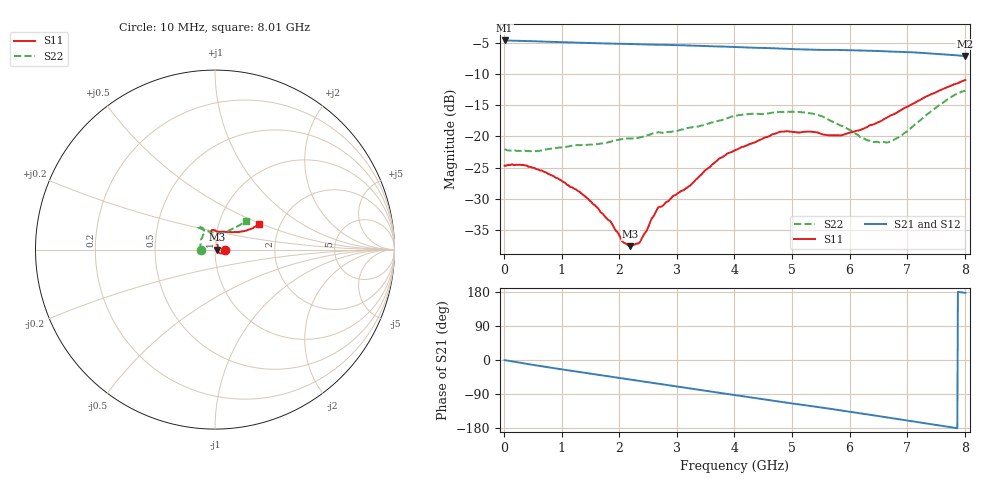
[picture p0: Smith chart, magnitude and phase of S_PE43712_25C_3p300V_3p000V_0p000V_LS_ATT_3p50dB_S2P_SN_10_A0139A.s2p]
! DEVICE ID: PE43712
! File Path: z:\PE43713\PE43713_CHAR_NOM_04292014\AMB\3p300\LS_ATT_3p50dB\PE43713_AMB_3p300V_3p000V_0p000V_LS_ATT_3p50dB_S2P_SN_10_A0139A.s2p
! Serial: 10
! Lot: A0139A
! Temp: 25C
! VDD: 3.300
! VSS: 0.000
! Control_Hi: 3.000
! Control_Lo: 0.000
! Attenuation Step: 3.50dB
! Port 1: RF1
! Port 2: RF2
! ThroughPath:1-2
! IDD: 0.0001469566
! ISS: -8.22e-008
#  Hz  S  RI  R  50
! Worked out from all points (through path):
!   801 points, 10 MHz to 8.01 GHz, reference 50 ohm
!   highest |S21| = -4.58 dB at 10 MHz (marker M1); lowest = -7.1 dB at 8 GHz (marker M2)
!   group delay of S21, straight-line fit = 62.7 ps
!   lowest |S11| = -37.6 dB at 2.19 GHz (marker M3), VSWR 1.03, Z = 51.3 - j0.093 ohm
!   |S11| at or under -10 dB: start of sweep to end of sweep
!   |S22| runs from -22.4 to -12.6 dB; largest |S21 - S12| = 0.0017
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1e7  0.0582 -0.000179  0.5901 -0.00314  0.59 -0.00291  -0.0785 0.000335
3.4e8  0.0575 -0.0121  0.5776 -0.0895  0.5772 -0.0881  -0.0762 0.00407
6.3e8  0.0501 -0.0183  0.557 -0.1586  0.5567 -0.1586  -0.0763 0.00902
9.6e8  0.0397 -0.0215  0.5236 -0.2302  0.5237 -0.2301  -0.0797 0.0161
1.35e9  0.0278 -0.0204  0.4756 -0.3041  0.4755 -0.3041  -0.0811 0.0261
1.85e9  0.018 -0.0102  0.4015 -0.3862  0.4015 -0.386  -0.0786 0.0451
2.07e9  0.0133 -0.00467  0.3646 -0.4175  0.3646 -0.4173  -0.079 0.0534
2.19e9  0.0131 -0.000906  0.3434 -0.4333  0.3434 -0.4329  -0.0768 0.0579
2.36e9  0.0126 0.00652  0.3116 -0.4535  0.3116 -0.4532  -0.0719 0.0665
2.68e9  0.0153 0.0221  0.2506 -0.4836  0.2506 -0.4836  -0.062 0.0885
3.22e9  0.00654 0.0395  0.1392 -0.5189  0.1394 -0.519  -0.0615 0.0999
3.72e9  0.00029 0.0653  0.0355 -0.527  0.0353 -0.5269  -0.0657 0.116
4.01e9  -0.00811 0.077  -0.0249 -0.5225  -0.0248 -0.5225  -0.0771 0.1242
4.79e9  -0.0199 0.1072  -0.1736 -0.4773  -0.1735 -0.4777  -0.0931 0.1268
5.35e9  -0.00668 0.1087  -0.264 -0.422  -0.2639 -0.4217  -0.0916 0.1222
5.86e9  0.024 0.0992  -0.3393 -0.3605  -0.3388 -0.3604  -0.0554 0.1081
6.32e9  0.0689 0.0988  -0.3941 -0.2887  -0.3932 -0.2885  -0.0139 0.0918
6.68e9  0.1068 0.0973  -0.4261 -0.2243  -0.4256 -0.2243  0.0209 0.0877
6.9e9  0.1309 0.0976  -0.4413 -0.1833  -0.4409 -0.1833  0.0436 0.0917
7.71e9  0.2174 0.124  -0.4525 -0.0279  -0.4523 -0.0283  0.1432 0.1406
8e9  0.2452 0.1401  -0.4415 0.0203  -0.441 0.0196  0.1704 0.1578
8.01e9  0.2461 0.1411  -0.4415 0.0217  -0.4408 0.0208  0.1713 0.1585
